| Texas Instruments Incorporated
| USB 3.0 Four Port Hub
| Marketing part#   Voltage Range   Package-type   Temperature
| TUSB8040PFP   2.97V - 3.465V   80-Pin pQFP   -40 to 105 C
| TUSB8040RKM   2.97V - 3.465V   100-Pin pQFP   -40 to 105 C
[IBIS Ver]   4.0
[File name]   tusb8040.ibs
[File Rev]   1.0
[Date]   12/07/2010
[Source]   Model built from TISPICE simulations at:
   Texas Instruments Incorporated.
   Analog-eLab, HPA
   12500 TI Blvd
   Dallas, TX -75243
   For Support e-mail: elab_scm_ibis@list.ti.com
[Notes]   Rev 1.0: 12/07/2010
   - Model based on tusb1310.ibs v1.1 09/14/2010 IBIS model.
   - Model generated from simulations in TISPICED
   - For USB2.0, models are included for HS, FS and LS modes
   - For USB3.0, models are included for SATA1, SATA2, No-De-Emphasis
   and De-Emphasis modes
   - USB2 and USB3 Models  matched to TISPICE.
   - C_comp although listed in numerical order of value are obtained from varying
   PVT conditions. For PVT conditions for each specific value refer the buffer
   description under respective [Model]. IBIS model user is responsible for using
   appropriate C_comp to simulate for Signal Integrity
   Where for TUSB8040
   Nom PVT:  Nominal process, Typ Temperature, Typ Voltage
   Slow PVT: Weak process, Max Temperature, Min Voltage
   Fast PVT: Strong process, Min Temperatire, Max Voltage
   - ignore warnings related to usb3_WODE, please do not correct this error
   as IBIS parser does not correct IV-VT mismatch with single set of V-T
   waveforms.
   - non-monotonic warnings related to usb2_LS_RC and usb2_LS_R buffers are
   as they are seen in TISPICE simualations
   - [Driver Schedule] is interpreted differently by each system level simulator
   , if usual setup with it does not give appropriate results, please
   tie the MAIN and BOOST buffers as per buffer timing description under
   [Driver Schedule] keyword. For example, using HSPICE, refer DE_hspice.sp
   in the correlation report
   - To test USB2/USB3 IBIS models using HSPICE look for spice set up files
   inside the TUSB8040 correlation report   \
   - Digital Buffer models are from SR60 standard cell library for TUSB8040
   - Non-Monotonic pulldown warnings related to digital buffers is per
   simulations
[Disclaimer] This product is designed as an aid for customers of Texas Instruments.
   No warranties, either expressed or implied, with respect to this third
   party software (if any) or with respect to its fitness for any
   particular purpose is claimed by Texas Instruments or the author. The
   software (if any) is provided solely on an "as is" basis. The entire
   risk as to its quality and performance is with the customer
[Copyright]   (C)Copyright 2010 Texas Instruments Incorporated.
   All rights reserved.
|   TUSB8040 PFP 80-pin pQFP
[Component]   TUSB8040PFP
[Manufacturer]  Texas Instruments Incorporated
[Package]   |80-pin PFP pQFP
|   typ   min   max
R_pkg   0.2389   0.0142   0.3346
L_pkg   3.3741nH   1.4298nH   4.8522nH
C_pkg   0.8499pF   0.7143pF   1.0609pF
[PIN]   signal_name   model_name   R_pin   L_pin   C_pin
1   VDD11   POWER   0.30413   4.521125nH   0.75199pF
2   USB_DN0_D_P   usb2   0.30924   3.077952nH   0.88517pF
3   USB_DN0_D_N   usb2   0.29228   2.818502nH   0.83867pF
4   VDD33   POWER   0.27754   4.089121nH   0.80467pF
5   VDD11   POWER   0.14229   3.592009nH   0.85747pF
6   USB_DN0_SSRX_P  RXP_N   0.25531   2.597727nH   0.78724pF
7   USB_DN0_SSRX_N  RXP_N   0.24475   2.442727nH   0.75922pF
8   USB_DN0_SSTX_P  usb3   0.23831   2.43116nH   0.75785pF
9   USB_DN0_SSTX_N  usb3   0.23245   2.34565nH   0.74929pF
10   VDD11   POWER   0.22865   3.387768nH   0.73322pF
11   VDD11   POWER   0.23954   3.514117nH   0.7686pF
12   USB_DN2_SSRX_P  RXP_N   0.23595   2.367264nH   0.76395pF
13   USB_DN2_SSRX_N  RXP_N   0.24363   2.476774nH   0.76606pF
14   USB_DN2_SSTX_P  usb3   0.25084   2.485487nH   0.77234pF
15   USB_DN2_SSTX_N  usb3   0.26282   2.659307nH   0.77764pF
16   VDD11   POWER   0.14731   3.710345nH   0.84651pF
17   USB_DN2_D_P   usb2   0.27768   2.731441nH   0.82584pF
18   USB_DN2_D_N   usb2   0.29279   2.917121nH   0.84433pF
19   VDD33   POWER   0.30971   4.51291nH   0.87029pF
20   VDD11   POWER   0.17259   4.852171nH   0.81335pF
21   VDD33   POWER   0.13268   3.844396nH   0.95243pF
22   HS   BC3340DSHYPBFZP18   0.24689   4.123684nH   1.0052pF
23   SS   BC3340DSHYPBFZP18   0.24379   3.996004nH   0.96623pF
24   HS_SUSPEND   BC3340DSHYPBFZP18   0.24221   3.894363nH   0.93222pF
25   SS_SUSPEND   BC3340DSHYPBFZP18   0.24305   3.818884nH   0.90481pF
26   VDD11   POWER   0.01498   1.522775nH   0.74735pF
27   JTAG_TCK   BC3340DSHYPBFZP18PD   0.23863   3.696742nH   0.86914pF
28   JTAG_TMS   BC3340DSHYPBFZP18PU   0.23718   3.640615nH   0.86049pF
29   JTAG_TDO   BC3340DSHYPBFZP18PD   0.23884   3.65016nH   0.84941pF
30   JTAG_RSTZ   IC33SHYPBFZP18PD   0.24292   3.697925nH   0.81516pF
31   JTAG_TDI   IC33SHYPBFZP18PU   0.25333   3.818604nH   0.82285pF
32   VDD11   POWER   0.0142   1.429796nH   0.71425pF
33   GRSTZ   IC33SHYPBFZP18PU   0.26123   3.919714nH   0.88825pF
34   SCL_SMBCLK   BC3340DSHYPBFZP18PD   0.27279   4.093598nH   0.90673pF
35   SDA_SMBDAT   BC3340DSHYPBFZP18PD   0.28586   4.279696nH   0.92621pF
36   SMBUSZ   IC33SHYPBFZP18PU   0.30032   4.486544nH   0.95748pF
37   VDD11   POWER   0.01575   1.614493nH   0.77262pF
38   VDD33   POWER   0.30223   4.598407nH   1.00915pF
39   PWRON0Z_BATEN0  BC3340DSHYPBFZP18PD   0.30334   4.664616nH   1.0136pF
40   OVERCUR0Z   IC33SHYPBFZP18PU   0.29425   4.590695nH   0.85471pF
41   FULLPWRMGMTZ_SMBA1 IC33SHYPBFZP18PU   0.32841   4.797447nH   0.79119pF
42   VDD11   POWER   0.33458   4.79462nH   0.88378pF
43   VDD33   POWER   0.31285   4.494757nH   0.86274pF
44   USM_DN3_D_N   usb2   0.29636   2.952481nH   0.81953pF
45   USB_DN3_D_P   usb2   0.28032   2.720481nH   0.79778pF
46   VDD11   POWER   0.27509   4.001721nH   0.79597pF
47   USB_DN3_SSRX_P  RXP_N   0.26131   2.630664nH   0.76831pF
48   USB_DN3_SSRX_N  RXP_N   0.24938   2.455334nH   0.76813pF
49   USB_DN3_SSTX_P  usb3   0.24258   2.459508nH   0.77065pF
50   USB_DN3_SSTX_N  usb3   0.23386   2.331198nH   0.74577pF
51   VDD11   POWER   0.23853   3.495964nH   0.7628pF
52   VDD11   POWER   0.12363   3.115186nH   0.8278pF
53   USB_DN1_SSRX_P  RXP_N   0.23295   2.347478nH   0.75231pF
54   USB_DN1_SSRX_N  RXP_N   0.23951   2.454708nH   0.75643pF
55   USB_DN1_SSTX_P  usb3   0.24574   2.457725nH   0.76995pF
56   USB_DN1_SSTX_N  usb3   0.25674   2.627125nH   0.77346pF
57   VDD11   POWER   0.144   3.699742nH   0.84612pF
58   VDD33   POWER   0.27939   4.097029nH   0.82422pF
59   USB_DN1_D_N   usb2   0.2952   2.856142nH   0.86651pF
60   USB_DN1_D_P   usb2   0.31144   3.139422nH   0.80644pF
61   VDD11   POWER   0.23575   4.046791nH   0.85053pF
62   VDD11   POWER   0.15435   4.490397nH   1.06093pF
63   USB_UP_SSTX_N   usb3   0.28343   3.014281nH   1.00172pF
64   USB_UP_SSTX_P   usb3   0.27667   2.841051nH   0.97048pF
65   USB_UP_SSRX_N   RXP_N   0.27173   2.833328nH   0.93864pF
66   USB_UP_SSRX_P   RXP_N   0.26036   2.650038nH   0.91537pF
67   VDD11   POWER   0.13284   3.42636nH   0.9549pF
68   VDD33   POWER   0.24664   3.731433nH   0.87998pF
69   USB_UP_D_N   usb2   0.24021   2.49803nH   0.86301pF
70   USB_UP_D_P   usb2   0.23588   2.44193nH   0.8281pF
71   VDD11   POWER   0.12394   3.17741nH   0.88997pF
72   VDD33   POWER   0.23427   3.578235nH   0.85368pF
73   USB_VBUS   NC   0.23423   3.587523nH   0.85314pF
74   XO   NC   0.2356   3.643268nH   0.88156pF
75   VSS_OSC   NC   0.23496   3.670547nH   0.88722pF
76   XI   NC   0.23697   3.732467nH   0.89892pF
77   VDD33   POWER   0.23689   3.802769nH   0.92301pF
78   USB_R1   NC   0.23554   3.870007nH   0.95365pF
79   VSS_R1RTN   GND   0.23667   3.974681nH   0.98832pF
80   VDD33   POWER   0.23835   4.077128nH   0.8651pF
[Diff_pin]   inv_pin   vdiff   tdelay_typ   tdelay_min   tdelay_max
2   3   880mV  NA NA NA| USB_DN0_DP/N
6   7   2200mV NA NA NA| USB_DN0_SSRXP/N
8   9   2200mV NA NA NA| USB_DN0_SSTXP/N
12   13   2200mV NA NA NA| USB_DN2_SSRXP/N
14   15   2200mV NA NA NA| USB_DN2_SSTXP/N
17   18   880mV  NA NA NA| USB_DN2_DP/M
45   44   880mV  NA NA NA| USB_DN3_DP/M
47   48   2200mV NA NA NA| USB_DN3_SSRXP/N
49   50   2200mV NA NA NA| USB_DN3_SSTXP/N
53   54   2200mV NA NA NA| USB_DN1_SSRXP/N
55   56   2200mV NA NA NA| USB_DN1_SSTXP/N
60   59   880mV  NA NA NA| USB_DN1_DP/N
64   63   2200mV NA NA NA| USB_UP_SSTXP/N
66   65   2200mV NA NA NA| USB_UP_SSRXP/N
70   69   880mV  NA NA NA| USB_UP_DP/N
[Pin Mapping] pulldown_ref pullup_ref gnd_clamp_ref power_clamp_ref |ext_ref
1   NC   VDD11BUS
2   VSSBUS   VDD33BUS   VSSBUS   VDD33BUS
3   VSSBUS   VDD33BUS   VSSBUS   VDD33BUS
4   NC   VDD33BUS
5   NC   VDD11BUS
6   NC   NC   VSSBUS   VDD11BUS
7   NC   NC   VSSBUS   VDD11BUS
8   VSSBUS   VDD11BUS
9   VSSBUS   VDD11BUS
10   NC   VDD11BUS
11   NC   VDD11BUS
12   NC   NC   VSSBUS   VDD11BUS
13   NC   NC   VSSBUS   VDD11BUS
14   VSSBUS   VDD11BUS
15   VSSBUS   VDD11BUS
16   NC   VDD11BUS
17   VSSBUS   VDD33BUS   VSSBUS   VDD33BUS
18   VSSBUS   VDD33BUS   VSSBUS   VDD33BUS
19   NC   VDD33BUS
20   NC   VDD11BUS
21   NC   VDD33BUS
22   VSSBUS   VDD33BUS   VSSBUS   VDD33BUS
23   VSSBUS   VDD33BUS   VSSBUS   VDD33BUS
24   VSSBUS   VDD33BUS   VSSBUS   VDD33BUS
25   VSSBUS   VDD33BUS   VSSBUS   VDD33BUS
26   NC   VDD11BUS
27   VSSBUS   VDD33BUS   VSSBUS   VDD33BUS
28   VSSBUS   VDD33BUS   VSSBUS   VDD33BUS
29   VSSBUS   VDD33BUS   VSSBUS   VDD33BUS
30   NC   NC   VSSBUS   VDD33BUS
31   NC   NC   VSSBUS   VDD33BUS
32   NC   VDD11BUS
33   NC   NC   VSSBUS   VDD33BUS
34   VSSBUS   VDD33BUS   VSSBUS   VDD33BUS
35   VSSBUS   VDD33BUS   VSSBUS   VDD33BUS
36   NC   NC   VSSBUS   VDD33BUS
37   NC   VDD11BUS
38   NC   VDD33BUS
39   VSSBUS   VDD33BUS   VSSBUS   VDD33BUS
40   NC   NC   VSSBUS   VDD33BUS
41   NC   NC   VSSBUS   VDD33BUS
42   NC   VDD11BUS
43   NC   VDD33BUS
44   VSSBUS   VDD33BUS   VSSBUS   VDD33BUS
45   VSSBUS   VDD33BUS   VSSBUS   VDD33BUS
46   NC   VDD11BUS
47   NC   NC   VSSBUS   VDD11BUS
48   NC   NC   VSSBUS   VDD11BUS
49   VSSBUS   VDD11BUS
50   VSSBUS   VDD11BUS
51   NC   VDD11BUS
52   NC   VDD11BUS
53   NC   NC   VSSBUS   VDD11BUS
54   NC   NC   VSSBUS   VDD11BUS
55   VSSBUS   VDD11BUS
56   VSSBUS   VDD11BUS
57   NC   VDD11BUS
58   NC   VDD33BUS
59   VSSBUS   VDD33BUS   VSSBUS   VDD33BUS
60   VSSBUS   VDD33BUS   VSSBUS   VDD33BUS
61   NC   VDD11BUS
62   NC   VDD11BUS
63   VSSBUS   VDD11BUS
64   VSSBUS   VDD11BUS
65   NC   NC   VSSBUS   VDD11BUS
66   NC   NC   VSSBUS   VDD11BUS
67   NC   VDD11BUS
68   NC   VDD33BUS
69   VSSBUS   VDD33BUS   VSSBUS   VDD33BUS
70   VSSBUS   VDD33BUS   VSSBUS   VDD33BUS
71   NC   VDD11BUS
72   NC   VDD33BUS
73   NC   NC
74   NC   NC
75   NC   NC
76   NC   NC
77   NC   VDD33BUS
78   NC   NC
79   VSSBUS   NC
80   NC   VDD33BUS
|   TUSB8040 RKM 100-pin pQFP
[Component]   TUSB8040RKM
[Manufacturer]  Texas Instruments Incorporated
[Package]   |100-pin RKM pQFP
|   typ   min   max
R_pkg   0.1422   0.0002   0.2301
L_pkg   1.6976nH   0.0002nH   2.9632nH
C_pkg   0.2522pF   0.0482pF   0.4093pF
[PIN]   signal_name   model_name   R_pin   L_pin   C_pin
1   USB_DN0_D_N   usb2   0.23013   2.200433nH   0.30484pF
2   USB_DN0_D_P   usb2   0.17472   1.315683nH   0.27153pF
3   VDD11   POWER   0.1069   2.606263nH   0.33854pF
4   VDD33   POWER   0.1613   2.001654nH   0.30361pF
5   USB_DN0_SSRX_P   RXP_N   0.19108   1.82297nH   0.2636pF
6   USB_DN0_SSRX_N   RXP_N   0.14017   1.01089nH   0.26536pF
7   USB_DN0_SSTX_P   usb3   0.17487   1.66702nH   0.2463pF
8   USB_DN0_SSTX_N   usb3   0.1259   0.8875nH   0.24578pF
9   VDD33   POWER   0.1565   1.946491nH   0.21039pF
10   NC   NC   0.00023   0.00023nH   0.10722pF
11   VDD11   POWER   0.15208   1.882559nH   0.2128pF
12   USB_DN2_SSRX_P   RXP_N   0.10432   0.729525nH   0.22088pF
13   USB_DN2_SSRX_N   RXP_N   0.1402   1.300895nH   0.19441pF
14   USB_DN2_SSTX_P   usb3   0.10231   0.703653nH   0.21241pF
15   USB_DN2_SSTX_N   usb3   0.14129   1.322373nH   0.1995pF
16   VDD11   POWER   0.05493   1.007025nH   0.26027pF
17   USB_DN2_D_P   usb2   0.14332   1.322836nH   0.19559pF
18   UDB_DN2_D_N   usb2   0.10919   0.777676nH   0.22728pF
19   VDD33   POWER   0.15253   1.888768nH   0.22428pF
20   VDD11   POWER   0.06664   1.179492nH   0.33718pF
21   HS_ALT0   NC   0.16053   2.005204nH   0.22487pF
22   HS_SUSPEND_ALT0   NC   0.12818   1.522705nH   0.25386pF
23   SS_ALT0   NC   0.18058   2.298702nH   0.26295pF
24   VDD11   POWER   0.07429   1.545232nH   0.25994pF
25   SS_SUSPEND_ALT0   NC   0.20192   2.613317nH   0.26017pF
26   VDD33   POWER   0.10711   2.430902nH   0.32791pF
27   JTAG_TCK   BC3340DSHYPBFZP18PD 0.19143   2.449617nH   0.27073pF
28   JTAG_TDO   BC3340DSHYPBFZP18PD 0.22542   2.963182nH   0.33222pF
29   JTAG_TMS   BC3340DSHYPBFZP18PU 0.17109   2.145479nH   0.32591pF
30   JTAG_RSTZ   IC33SHYPBFZP18PD   0.20459   2.652516nH   0.28278pF
31   JTAG_TDI   IC33SHYPBFZP18PU   0.15811   1.953752nH   0.2918pF
32   LPWRMGMTZ_SMBA1_ALT0  NC   0.19069   2.44611nH   0.24476pF
33   VDD11   POWER   0.08118   1.535864nH   0.37426pF
34   GRSTN   IC33SHYPBFZP18PU   0.18574   2.372803nH   0.2695pF
35   SCL_SMBCLK   BC3340DSHYPBFZP18PD 0.14279   1.729825nH   0.26132pF
36   SDA_SMBDAT   BC3340DSHYPBFZP18PD 0.17825   2.261556nH   0.23914pF
37   SMBUSZ   IC33SHYPBFZP18PU   0.13768   1.654861nH   0.24699pF
38   VPP   POWER   0.08831   1.857087nH   0.27648pF
39   PWRON0Z_BATEN0   BC3340DSHYPBFZP18PD 0.14276   1.729082nH   0.25184pF
40   PWRON0Z_BATEN1   BC3340DSHYPBFZP18PD 0.17729   2.247144nH   0.24118pF
41   PWRON0Z_BATEN2   BC3340DSHYPBFZP18PD 0.13767   1.654629nH   0.25418pF
42   PWRON0Z_BATEN3   BC3340DSHYPBFZP18PD 0.1761   2.228798nH   0.22336pF
43   OVERCUR0Z_ALT0   IC33SHYPBFZP18PU   0.13713   1.646992nH   0.23447pF
44   OVERCUR1Z   IC33SHYPBFZP18PU   0.17737   2.247003nH   0.23742pF
45   OVERCUR2Z   IC33SHYPBFZP18PU   0.13987   1.68547nH   0.25441pF
46   OVERCUR23Z   IC33SHYPBFZP18PU   0.18389   2.341892nH   0.24634pF
47   LEDA0Z_RMBL0   NC   0.14792   1.80172nH   0.27129pF
48   LEDG0Z_USED0   NC   0.19517   2.507356nH   0.26567pF
49   VDD33   POWER   0.08018   1.642417nH   0.31015pF
50   VDD11   POWER   0.10335   1.991128nH   0.3687pF
51   LEDG1Z_USED1   NC   0.20957   2.722231nH   0.26784pF
52   LEDA1Z_RMBL1   NC   0.15382   1.890754nH   0.23828pF
53   LEDG2Z_USED2   NC   0.20189   2.606131nH   0.27387pF
54   LEDA2Z_RMBL2   NC   0.14881   1.813813nH   0.26647pF
55   LEDA3Z_RMBL3   NC   0.1787   2.263132nH   0.30262pF
56   VDD11   POWER   0.1412   1.701659nH   0.31163pF
57   LEDG3Z_USED3   NC   0.15951   1.981471nH   0.21983pF
58   VDD33   POWER   0.11942   1.388107nH   0.23762pF
59   USB_DN3_D_N   usb2   0.14993   1.406989nH   0.21069pF
60   USB_DN3_D_P   usb2   0.10779   0.738449nH   0.21893pF
61   VDD11   POWER   0.14456   1.763485nH   0.20239pF
62   USB_DN3_SSRX_P   RXP_N   0.10413   0.722207nH   0.21543pF
63   USB_DN3_SSRX_N   RXP_N   0.14015   1.294387nH   0.19631pF
64   USB_DN3_SSTX_P   usb3   0.10233   0.697685nH   0.21824pF
65   USB_DN3_SSTX_N   usb3   0.14142   1.317645nH   0.19505pF
66   NC   NC   0.00023   0.00023nH   0.10722pF
67   VDD11   POWER   0.07608   1.694209nH   0.23591pF
68   USB_DN1_SSRX_P   RXP_N   0.11696   0.816296nH   0.23365pF
69   USB_DN1_SSRX_N   RXP_N   0.16083   1.513256nH   0.23026pF
70   USB_DN1_SSTX_P   usb3   0.12894   0.920449nH   0.26242pF
71   USB_DN1_SSTX_N   usb3   0.17424   1.641779nH   0.26257pF
72   VDD33   POWER   0.14287   1.727204nH   0.28351pF
73   VDD11   POWER   0.10007   2.238144nH   0.34692pF
74   USB_DN1_D_P   usb2   0.15826   1.160928nH   0.25211pF
75   USB_DN1_D_N   usb2   0.21427   2.049538nH   0.28924pF
76   NC   NC   0.00027   0.007422nH   0.04823pF
77   PORTINDZ_SMBA3   NC   0.1771   2.230307nH   0.25226pF
78   GANGED_SMBA2   NC   0.20968   2.722231nH   0.26015pF
79   VDD11   POWER   0.09336   1.808627nH   0.40927pF
80   USB_UP_SSTX_N   usb3   0.21099   1.98462nH   0.30894pF
81   USB_UP_SSTX_P   usb3   0.16467   1.24263nH   0.304pF
82   USB_UP_SSRX_N   usb2   0.19826   1.861779nH   0.27371pF
83   USB_UP_SSRX_P   usb2   0.15353   1.145609nH   0.2759pF
84   VDD11   POWER   0.09367   2.00144nH   0.30509pF
85   VDD33   POWER   0.16692   2.078161nH   0.2957pF
86   USB_UP_D_N   usb2   0.18045   1.685712nH   0.25847pF
87   USB_UP_D_P   usb2   0.13922   1.025802nH   0.26399pF
88   VDD11   POWER   0.0891   1.867795nH   0.30383pF
89   VDD33   POWER   0.13807   1.659409nH   0.24939pF
90   USB_VBUS   NC   0.17716   2.243928nH   0.2138pF
91   XO   NC   0.14333   1.734557nH   0.24981pF
92   VSSOSC   NC   0.17718   2.244153nH   0.24243pF
93   XI   NC   0.13792   1.657061nH   0.25942pF
94   VDD33   POWER   0.17612   2.22951nH   0.23227pF
95   USB_R1   NC   0.13754   1.652921nH   0.25057pF
96   VSS_R1EXTRTN   GND   0.17962   2.281834nH   0.22509pF
97   NC   NC   0.00023   0.00023nH   0.10506pF
98   NC   NC   0.00027   0.005912nH   0.0565pF
99   VDD33   POWER   0.15556   1.921801nH   0.23189pF
100   VDD11   POWER   0.20529   2.662711nH   0.26088pF
[Diff_pin]   inv_pin   vdiff   tdelay_typ   tdelay_min   tdelay_max
2   1   880mV  NA NA NA| USB_DP/DM_DN0
5   6   2200mV NA NA NA| USB_SSRX_P/N_DN0
7   8   2200mV NA NA NA| USB_SSTX_P/N_DN0
12   13   2200mV NA NA NA| USB_SSRX_P/N_DN2
14   15   2200mV NA NA NA| USB_SSTX_P/N_DN2
17   18   880mV  NA NA NA| USB_DN2_DP/N
62   63   2200mV NA NA NA| USB_DN3_SSRXP/N
64   65   2200mV NA NA NA| USB_DN3_SSTXP/N
68   69   2200mV NA NA NA| USB_DN1_SSRXP/N
70   71   2200mV NA NA NA| USB_DN1_SSTXP/N
74   75   880mV  NA NA NA| USB_DN1_DP/N
81   80   2200mV NA NA NA| USB_UP_SSTXP/N
83   82   2200mV NA NA NA| USB_UP_SSRXP/N
87   86   880mV  NA NA NA| USB_UP_DP/N
[Pin Mapping] pulldown_ref pullup_ref gnd_clamp_ref power_clamp_ref |ext_ref
1   VSSBUS  VDD33BUS   VSSBUS   VDD33BUS
2   VSSBUS  VDD33BUS   VSSBUS   VDD33BUS
3   NC   VDD11BUS
4   NC   VDD11BUS
5   NC   NC   VSSBUS   VDD11BUS
6   NC   NC   VSSBUS   VDD11BUS
7   VSSBUS  VDD11BUS
8   VSSBUS  VDD11BUS
9   NC   VDD33BUS
10   NC   NC
11   NC   VDD11BUS
12   NC   NC   VSSBUS   VDD11BUS
13   NC   NC   VSSBUS   VDD11BUS
14   VSSBUS  VDD11BUS
15   VSSBUS  VDD11BUS
16   NC   VDD11BUS
17   VSSBUS  VDD33BUS   VSSBUS   VDD33BUS
18   VSSBUS  VDD33BUS   VSSBUS   VDD33BUS
19   NC   VDD33BUS
20   NC   VDD11BUS
21   NC   NC
22   NC   NC
23   NC   NC
24   NC   VDD11BUS
25   NC   NC
26   NC   VDD33BUS
27   VSSBUS  VDD33BUS   VSSBUS   VDD33BUS
28   VSSBUS  VDD33BUS   VSSBUS   VDD33BUS
29   VSSBUS  VDD33BUS   VSSBUS   VDD33BUS
30   NC   NC   VSSBUS   VDD33BUS
31   NC   NC   VSSBUS   VDD33BUS
32   NC   NC
33   NC   VDD11BUS
34   NC   NC   VSSBUS   VDD33BUS
35   VSSBUS  VDD33BUS   VSSBUS   VDD33BUS
36   VSSBUS  VDD33BUS   VSSBUS   VDD33BUS
37   NC   NC   VSSBUS   VDD33BUS
38   NC   VPPBUS
39   VSSBUS  VDD33BUS   VSSBUS   VDD33BUS
40   VSSBUS  VDD33BUS   VSSBUS   VDD33BUS
41   VSSBUS  VDD33BUS   VSSBUS   VDD33BUS
42   VSSBUS  VDD33BUS   VSSBUS   VDD33BUS
43   NC   NC   VSSBUS   VDD33BUS
44   NC   NC   VSSBUS   VDD33BUS
45   NC   NC   VSSBUS   VDD33BUS
46   NC   NC   VSSBUS   VDD33BUS
47   NC   NC
48   NC   NC
49   NC   VDD33BUS
50   NC   VDD11BUS
51   NC   NC
52   NC   NC
53   NC   NC
54   NC   NC
55   NC   NC
56   NC   VDD11BUS
57   NC   NC
58   NC   VDD33BUS
59   VSSBUS  VDD33BUS   VSSBUS   VDD33BUS
60   VSSBUS  VDD33BUS   VSSBUS   VDD33BUS
61   NC   VDD33BUS
62   NC   NC   VSSBUS   VDD33BUS
63   NC   NC   VSSBUS   VDD33BUS
64   VSSBUS  VDD11BUS
65   VSSBUS  VDD11BUS
66   NC   NC
67   NC   VDD11BUS
68   NC   NC   VSSBUS   VDD11BUS
69   NC   NC   VSSBUS   VDD11BUS
70   VSSBUS  VDD11BUS
71   VSSBUS  VDD11BUS
72   NC   VDD33BUS
73   NC   VDD11BUS
74   VSSBUS  VDD33BUS   VSSBUS   VDD33BUS
75   VSSBUS  VDD33BUS   VSSBUS   VDD33BUS
76   NC   NC
77   NC   NC
78   NC   NC
79   NC   VDD11BUS
80   NC   NC   VSSBUS  VDD11BUS
81   NC   NC   VSSBUS  VDD11BUS
82   VSSBUS  VDD11BUS
83   VSSBUS  VDD11BUS
84   NC   VDD11BUS
85   NC   VDD33BUS
86   VSSBUS  VDD33BUS   VSSBUS  VDD33BUS
87   VSSBUS  VDD33BUS   VSSBUS  VDD33BUS
88   NC   VDD11BUS
89   NC   VDD33BUS
90   NC   NC
91   NC   NC
92   NC   NC
93   NC   NC
94   NC   VDD33BUS
95   NC   NC
96   VSSBUS  NC
97   NC   NC
98   NC   NC
99   NC   VDD33BUS
100  NC   VDD11BUS
[Model Selector] usb2
usb2_HS_R   USB 2.0 High Speed mode, for DP/DM pin 240MHz
usb2_HS_RC   USB 2.0 High Speed mode, for DP/DM pin 240MHz, with Cfixture
usb2_FS_R   USB 2.0 Fast Speed mode, for DP/DM pin 6MHz
usb2_FS_RC   USB 2.0 Fast Speed mode, for DP/DM pin 6MHz, with Cfixture
usb2_LS_RC   USB 2.0 Low  Speed mode, for DP/DM pin 750kHz, with Cfixture
usb2_LS_R   USB 2.0 Low  Speed mode, for DP/DM pin 750kHz
[Model Selector] usb3
usb3_DE   USB 3.0 De-Emphasis mode, best at 1.25GHz
usb3_WODE   USB 3.0 No De-Emphasis mode, for SSTXP/N 2.5GHz
usb3_SATA1   USB 3.0 SATA1 mode, for SSTXP/N 750MHz
usb3_SATA2   USB 3.0 SATA2 mode, for SSTXP/N 1.5GHz
pcie_GEN2   PCI-E 2.5GHz  GEN2 model
pcie_GEN1   PCI-E 1.25GHz GEN1 model
[Model Selector] BC3340DSHYPBFZP18
HYPBFZP18_PI_5P_3P3 BUFFER WITHOUT PULLUP/PULLDOWN & 5% VDDS TOLERANCE
HYPBFZP18_PI_10P_3P3 BUFFER WITHOUT PULLUP/PULLDOWN & 10% VDDS TOLERANCE
[Model Selector] BC3340DSHYPBFZP18PU
FZP18_PU_PI_5P_3P3 BUFFER WITH WEAK PULLUP & 5% VDDS TOLERANCE
FZP18_PU_PI_10P_3P3 BUFFER WITH WEAK PULLUP & 10% VDDS TOLERANCE
[Model Selector] BC3340DSHYPBFZP18PD
FZP18_PD_PI_5P_3P3 BUFFER WITH WEAK PULLDOWN & 5% VDDS TOLERANCE
FZP18_PD_PI_10P_3P3 BUFFER WITH WEAK PULLDOWN & 10% VDDS TOLERANCE
[Model Selector] IC33SHYPBFZP18
C33SHYPBFZP18_10P BUFFER WITHOUT PULLUP/PULLDOWN & 10% VDDS TOLERANCE
C33SHYPBFZP18_5P  BUFFER WITHOUT PULLUP/PULLDOWN & 5% VDDS TOLERANCE
[Model Selector] IC33SHYPBFZP18PD
YPBFZP18_PD_5P BUFFER with WEAK PULLDOWN & 5% VDDS TOLERANCE
YPBFZP18_PD_10P BUFFER with WEAK PULLDOWN & 5% VDDS TOLERANCE
[Model Selector] IC33SHYPBFZP18PU
PBFZP18_PU_5P BUFFER with WEAK PULLUP & 5% VDDS TOLERANCE
PBFZP18_PU_10P BUFFER with WEAK PULLUP & 10% VDDS TOLERANCE
|USB 3.0 De-Emphasis mode, for SSTXP/SSTXN pins 2.5Gbps(1.25GHz to De-Emphasis)
[Model]   usb3_DE
Model_type   Output
Vmeas = 1.1
Vref = 1.1
Rref = 50
|   typ   min   max
|   (TYP PVT)   (Fast PVT) (Slow PVT)
C_comp   0pF   0pF   0pF
[Driver Schedule]
| Model_name   Rise_on_dly Rise_off_dly Fall_on_dly Fall_off_dly
usb3_de_MAIN   0.0nS   0.4ns   0   0.4ns
usb3_de_BOOST   0.0nS   0.2nS   0   0.2nS
[Voltage Range]   1.1   0.99   1.155
[Temperature Range]   27   105   -40
[Pullup Reference]   1.1   0.99   1.155
[Pulldown Reference]   0   0   0
[Power Clamp Reference]   1.1   0.99   1.155
[GND Clamp Reference]   0   0   0
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[Ramp]
R_load = 50
|   typ   min   max
dV/dt_r   0.972315/1.549e-011   0.988218/1.8606e-011   0.957162/1.40763e-011
dV/dt_f   0.972312/7.7916e-012   0.988183/1.21282e-011  0.957081/6.00194e-012
|PCIE GEN2 De-Emphasis mode, for SSTXP/SSTXN pins 5Gbps(2.5GHz to De-Emphasis)
[Model]   pcie_GEN2
Model_type   Output
Vmeas = 1.1
Vref = 1.1
Rref = 50
|   typ   min   max
|   (TYP PVT)   (Fast PVT) (Slow PVT)
C_comp   0pF   0pF   0pF
[Driver Schedule]
| Model_name   Rise_on_dly Rise_off_dly Fall_on_dly Fall_off_dly
usb3_de_MAIN   0.0nS   0.4ns   0   0.4ns
usb3_de_BOOST   0.0nS   0.2nS   0   0.2nS
[Voltage Range]   1.1   0.99   1.155
[Temperature Range]   27   105   -40
[Pullup Reference]   1.1   0.99   1.155
[Pulldown Reference]   0   0   0
[Power Clamp Reference]   1.1   0.99   1.155
[GND Clamp Reference]   0   0   0
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[Ramp]
R_load = 50
|   typ   min   max
dV/dt_r   0.972315/1.549e-011   0.988218/1.8606e-011   0.957162/1.40763e-011
dV/dt_f   0.972312/7.7916e-012   0.988183/1.21282e-011  0.957081/6.00194e-012
|PCIE GEN1 De-Emphasis mode, for SSTXP/SSTXN pins 2.5Gbps(1.25GHz to De-Emphasis)
[Model]   pcie_GEN1
Model_type   Output
Vmeas = 1.1
Vref = 1.1
Rref = 50
|   typ   min   max
|   (TYP PVT)   (Fast PVT) (Slow PVT)
C_comp   0pF   0pF   0pF
[Driver Schedule]
| Model_name   Rise_on_dly Rise_off_dly Fall_on_dly Fall_off_dly
usb3_de_MAIN   0.0nS   0.8ns   0   0.8ns
usb3_de_BOOST   0.0nS   0.4nS   0   0.4nS
[Voltage Range]   1.1   0.99   1.155
[Temperature Range]   27   105   -40
[Pullup Reference]   1.1   0.99   1.155
[Pulldown Reference]   0   0   0
[Power Clamp Reference]   1.1   0.99   1.155
[GND Clamp Reference]   0   0   0
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[Ramp]
R_load = 50
|   typ   min   max
dV/dt_r   0.972315/1.549e-011   0.988218/1.8606e-011   0.957162/1.40763e-011
dV/dt_f   0.972312/7.7916e-012   0.988183/1.21282e-011  0.957081/6.00194e-012
| Models and submodels in the file (27): RXP_N (Input), usb2_FS_R (I/O), usb2_FS_RC (I/O), usb2_HS_R (I/O), usb2_HS_RC (I/O), usb2_LS_R (I/O), usb2_LS_RC (I/O), usb3_WODE (Output), usb3_SATA1 (Output), usb3_SATA2 (Output), usb3_DE (Output), usb3_de_MAIN (Output), usb3_de_BOOST (Open_drain), pcie_GEN2 (Output), pcie_GEN1 (Output), HYPBFZP18_PI_5P_3P3 (I/O), HYPBFZP18_PI_10P_3P3 (I/O), FZP18_PU_PI_5P_3P3 (I/O), FZP18_PU_PI_10P_3P3 (I/O), FZP18_PD_PI_5P_3P3 (I/O), FZP18_PD_PI_10P_3P3 (I/O), YPBFZP18_PD_10P (Input), PBFZP18_PU_10P (Input), C33SHYPBFZP18_10P (Input), YPBFZP18_PD_5P (Input), PBFZP18_PU_5P (Input), C33SHYPBFZP18_5P (Input)
